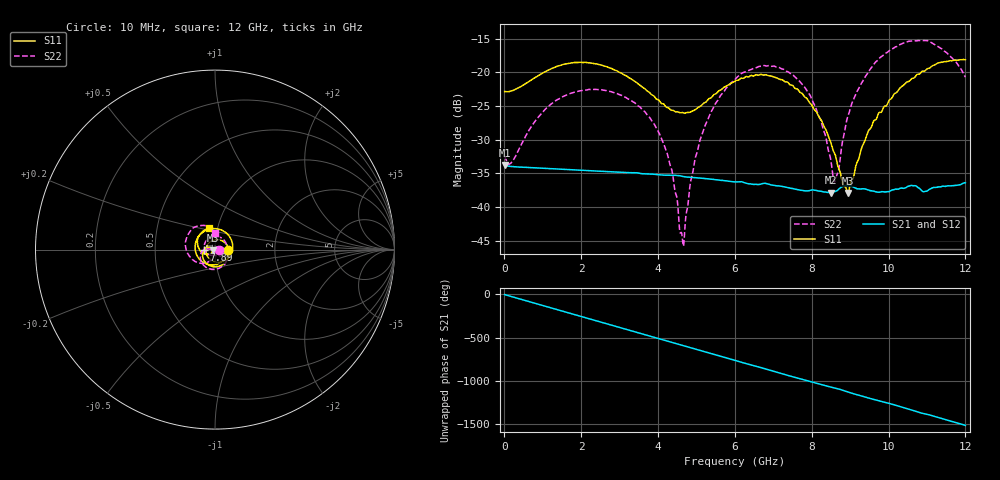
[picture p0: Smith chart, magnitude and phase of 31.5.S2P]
!Agilent Technologies,E5071C,MY46316741,A.11.02
!Date: Fri Apr 15 15:50:41 2022
!Data & Calibration Information:
!Freq	S11:SOLT2(ON)	S21:SOLT2(ON)	S12:SOLT2(ON)	S22:SOLT2(ON)
!PortZ  Port1:50+j0  Port2:50+j0
!Above PortZ is port z conversion or system Z0 setting when saving the data.
!When reading, reference impedance value at option line is always used.
# Hz S dB R 50
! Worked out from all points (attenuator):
!   1200 points, 10 MHz to 12 GHz, reference 50 ohm
!   highest |S21| = -33.78 dB at 10 MHz (marker M1); lowest = -37.9 dB at 8.51 GHz (marker M2)
!   lowest |S11| = -38.0 dB at 8.95 GHz (marker M3), VSWR 1.03, Z = 48.8 - j0.315 ohm
!   |S11| at or under -10 dB: start of sweep to end of sweep
!   |S22| runs from -45.8 to -15.3 dB; largest |S21 - S12| = 0.00016
!   S11 on the Smith chart (normalised r, x): 10 MHz: 1.15, -0.00; 7.89 GHz: 0.88, -0.01; 12 GHz: 0.91, +0.22
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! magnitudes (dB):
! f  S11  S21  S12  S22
! 10 MHz  -22.9  -33.8  -33.8  -32.4
! 200 MHz  -22.8  -34.0  -34.0  -33.3
! 1.16 GHz  -19.7  -34.3  -34.3  -25.0
! 2.01 GHz  -18.5  -34.6  -34.6  -22.7
! 3.22 GHz  -20.7  -34.9  -34.9  -24.0
! 4.01 GHz  -24.1  -35.2  -35.2  -28.8
! 4.34 GHz  -25.6  -35.3  -35.3  -34.2
! 4.63 GHz  -26.0  -35.5  -35.5  -44.4
! 4.9 GHz  -25.8  -35.6  -35.6  -35.1
! 5.15 GHz  -24.8  -35.8  -35.8  -29.3
! 6.01 GHz  -21.3  -36.3  -36.3  -21.1
! 7.02 GHz  -20.7  -36.8  -36.8  -19.1
! 7.89 GHz  -24.0  -37.6  -37.6  -22.9
! 8.01 GHz  -25.0  -37.5  -37.5  -24.1
! 8.31 GHz  -27.9  -37.8  -37.8  -28.7
! 8.51 GHz  -30.7  -37.9  -37.9  -33.5
! 8.65 GHz  -33.1  -37.6  -37.6  -35.4
! 8.95 GHz  -38.0  -36.9  -36.9  -26.4
! 9.46 GHz  -29.0  -37.5  -37.4  -20.1
! 10.01 GHz  -24.2  -37.7  -37.7  -16.9
! 11.03 GHz  -19.5  -37.5  -37.6  -15.3
! 12 GHz  -18.2  -36.4  -36.4  -20.7
